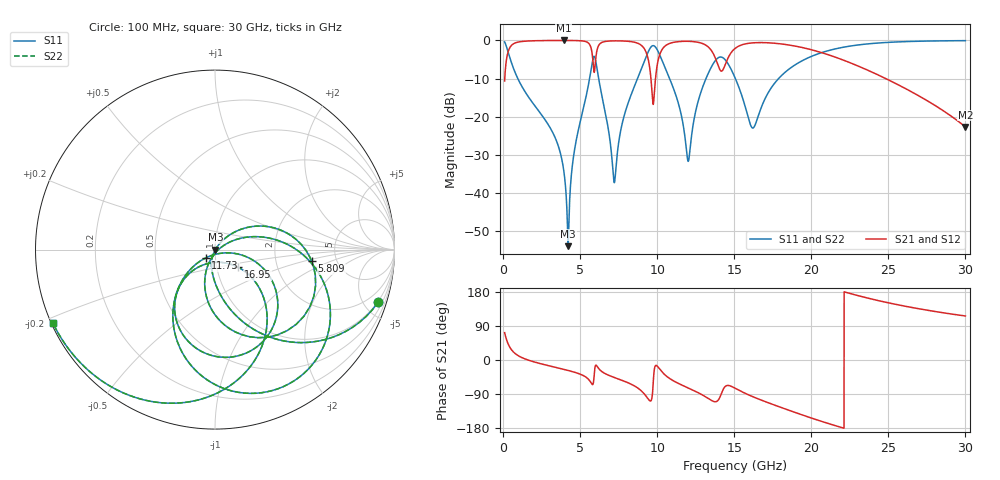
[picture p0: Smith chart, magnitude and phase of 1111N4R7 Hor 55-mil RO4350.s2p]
# GHz S MA R 50
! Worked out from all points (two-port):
!   3201 points, 100 MHz to 30 GHz, reference 50 ohm
!   highest |S21| = -0.02 dB at 3.931 GHz (marker M1); lowest = -22.7 dB at 30 GHz (marker M2)
!   |S21| within 3 dB of the highest: 323.8 MHz to 5.763 GHz (5.439 GHz wide, 179 % of centre); 14.84 GHz to 20.51 GHz (5.676 GHz wide, 32.1 % of centre)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
!   lowest |S11| = -53.9 dB at 4.221 GHz (marker M3), VSWR 1.00, Z = 50.2 - j0.0937 ohm
!   |S11| at or under -10 dB: 956.2 MHz to 5.613 GHz (4.656 GHz wide, 142 % of centre); 6.203 GHz to 8.723 GHz (2.52 GHz wide, 33.8 % of centre); 15.07 GHz to 17.88 GHz (2.804 GHz wide, 17 % of centre)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
!   |S22| runs from -53.9 to -0.1 dB; largest |S21 - S12| = 0
!   S11 on the Smith chart (normalised r, x): 100 MHz: 0.93, -6.26; 5.809 GHz: 3.26, -0.60; 11.73 GHz: 0.90, -0.08; 16.95 GHz: 1.27, -0.26; 30 GHz: 0.00, -0.22
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0.1  0.9557 -17.8  0.2941 72.2  0.2941 72.2  0.9557 -17.8
0.959625  0.3152 -77.9  0.9484 12.0  0.9484 12.0  0.3152 -77.9
3.930938  0.02016 -110.1  0.9978 -24.5  0.9978 -24.5  0.02016 -110.1
4.220594  0.002014 -27.6  0.9975 -27.5  0.9975 -27.5  0.002014 -27.6
5.089563  0.1013 46.5  0.986 -38.8  0.986 -38.8  0.1013 46.5
5.809031  0.5433 -6.9  0.5992 -65.0  0.5992 -65.0  0.5433 -6.9
6.257531  0.2739 -99.6  0.8911 -24.9  0.8911 -24.9  0.2739 -99.6
7.219938  0.01366 -42.8  0.9856 -46.2  0.9856 -46.2  0.01366 -42.8
8.808375  0.3493 8.7  0.9039 -75.9  0.9039 -75.9  0.3493 8.7
9.44375  0.727 -27.9  0.535 -104.3  0.535 -104.3  0.727 -27.9
9.74275  0.854 -61.0  0.1449 -60.9  0.1449 -60.9  0.854 -61.0
10.06978  0.7095 -95.7  0.5572 -19.2  0.5572 -19.2  0.7095 -95.7
11.73297  0.06844 -138.0  0.9727 -68.6  0.9727 -68.6  0.06844 -138.0
12.05066  0.02733 -59.5  0.9723 -74.4  0.9723 -74.4  0.02733 -59.5
12.72341  0.177 -12.7  0.9376 -87.5  0.9376 -87.5  0.177 -12.7
13.84466  0.5651 -59.1  0.539 -109.6  0.539 -109.6  0.5651 -59.1
15.05  0.3247 -131.1  0.7827 -74.3  0.7827 -74.3  0.3247 -131.1
16.16191  0.07163 -93.2  0.9267 -96.1  0.9267 -96.1  0.07163 -93.2
16.94678  0.1635 -37.2  0.9344 -108.8  0.9344 -108.8  0.1635 -37.2
20.03956  0.6209 -66.5  0.7511 -153.6  0.7511 -153.6  0.6209 -66.5
25.01978  0.9427 -120.7  0.3028 150.7  0.3028 150.7  0.9427 -120.7
30  0.9918 -155.7  0.07346 116.1  0.07346 116.1  0.9918 -155.7
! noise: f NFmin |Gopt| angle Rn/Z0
0.1  0.001181  0.8519  3.249  0.0017
3.417  0.009034  0.4482  23.4  0.002633
6.743  0.05019  0.7667  43.41  0.03788
10.06  0.2289  0.9195  63.07  0.4571
13.39  0.19  0.8766  81.04  0.1929
16.7  0.1274  0.7851  98.45  0.053
20.03  0.1163  0.7333  112.8  0.02805
23.35  0.1527  0.7737  126.6  0.02962
26.67  0.2509  0.8539  141.6  0.04175
30  0.577  0.9354  157.6  0.0778
